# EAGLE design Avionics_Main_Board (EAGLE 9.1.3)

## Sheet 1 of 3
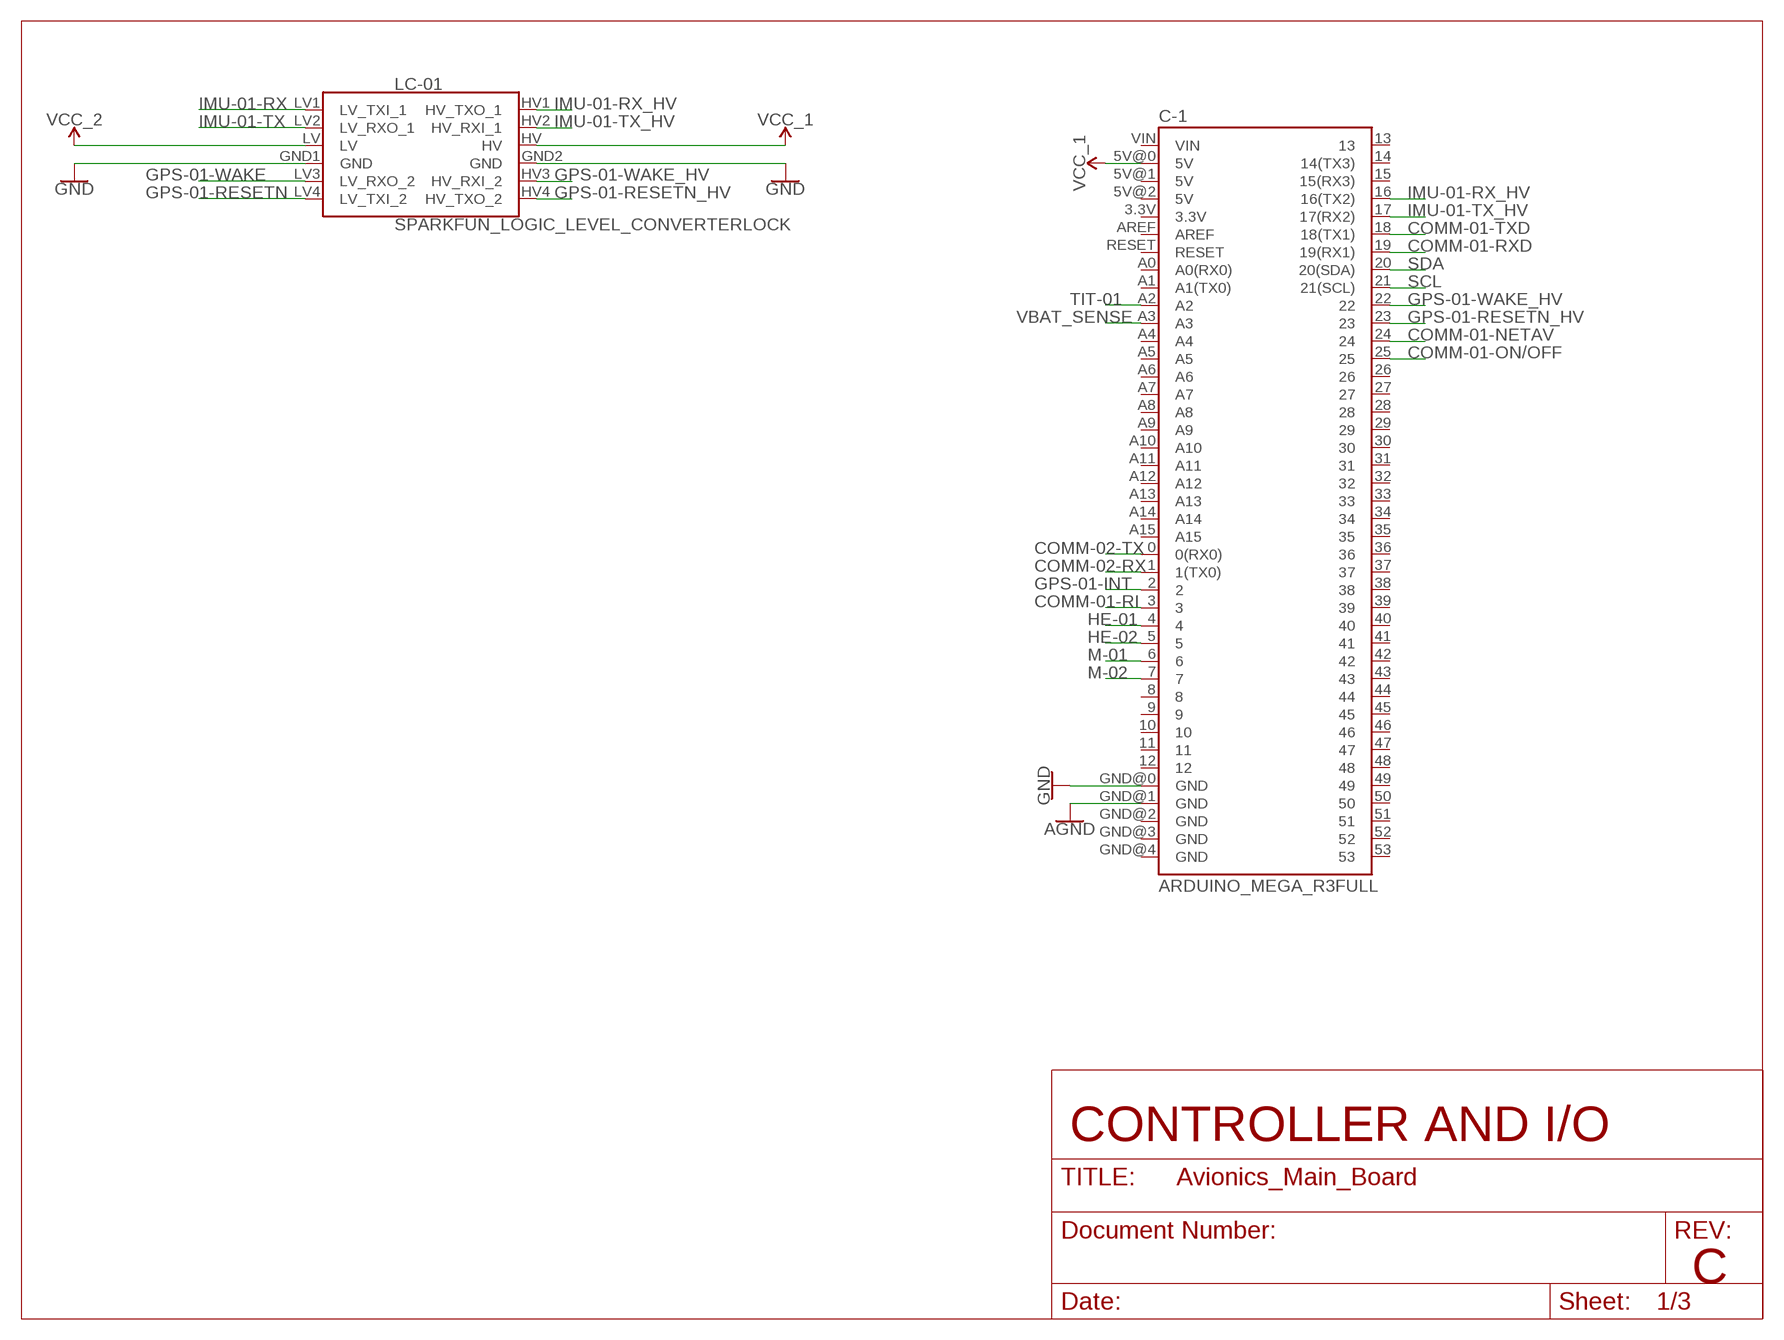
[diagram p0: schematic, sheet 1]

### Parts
C-1  ARDUINO_MEGA_R3FULL  [ARDUINO_MEGA]
LC-01  SPARKFUN_LOGIC_LEVEL_CONVERTERLOCK  [SPARKFUN_LOGIC_LEVEL_CONVERTER_LOCK]

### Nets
AGND: C-1.GND@1(GND) ; also sheet 3
COMM-01-NETAV: C-1.24 ; also sheet 3
COMM-01-ON/OFF: C-1.25 ; also sheet 3
COMM-01-RI: C-1.3 ; also sheet 3
COMM-01-RXD: C-1.19(19(RX1)) ; also sheet 3
COMM-01-TXD: C-1.18(18(TX1)) ; also sheet 3
COMM-02-RX: C-1.1(1(TX0)) ; also sheet 3
COMM-02-TX: C-1.0(0(RX0)) ; also sheet 3
GND: C-1.GND@0(GND) LC-01.GND1(GND) LC-01.GND2(GND) ; also sheet 2,3
GPS-01-INT: C-1.2 ; also sheet 3
GPS-01-RESETN: LC-01.LV4(LV_TXI_2) ; also sheet 3
GPS-01-RESETN_HV: C-1.23 LC-01.HV4(HV_TXO_2)
GPS-01-WAKE: LC-01.LV3(LV_RXO_2) ; also sheet 3
GPS-01-WAKE_HV: C-1.22 LC-01.HV3(HV_RXI_2)
HE-01: C-1.4 ; also sheet 2
HE-02: C-1.5 ; also sheet 2
IMU-01-RX: LC-01.LV1(LV_TXI_1) ; also sheet 3
IMU-01-RX_HV: C-1.16(16(TX2)) LC-01.HV1(HV_TXO_1)
IMU-01-TX: LC-01.LV2(LV_RXO_1) ; also sheet 3
IMU-01-TX_HV: C-1.17(17(RX2)) LC-01.HV2(HV_RXI_1)
M-01: C-1.6 ; also sheet 2
M-02: C-1.7 ; also sheet 2
SCL: C-1.21(21(SCL)) ; also sheet 3
SDA: C-1.20(20(SDA)) ; also sheet 3
TIT-01: C-1.A2 ; also sheet 3
VBAT_SENSE: C-1.A3 ; also sheet 3
VCC_1 [power]: C-1.5V@0(5V) LC-01.HV ; also sheet 2,3
VCC_2 [power]: LC-01.LV ; also sheet 2,3
Unconnected: C-1.3.3V C-1.5V@1(5V) C-1.5V@2(5V) C-1.8 C-1.9 C-1.10 C-1.11 C-1.12 C-1.13 C-1.14(14(TX3)) C-1.15(15(RX3)) C-1.26 C-1.27 C-1.28 C-1.29 C-1.30 C-1.31 C-1.32 C-1.33 C-1.34 C-1.35 C-1.36 C-1.37 C-1.38 C-1.39 C-1.40 C-1.41 C-1.42 C-1.43 C-1.44 C-1.45 C-1.46 C-1.47 C-1.48 C-1.49 C-1.50 C-1.51 C-1.52 C-1.53 C-1.A0(A0(RX0)) C-1.A1(A1(TX0)) C-1.A4 C-1.A5 C-1.A6 C-1.A7 C-1.A8 C-1.A9 C-1.A10 C-1.A11 C-1.A12 C-1.A13 C-1.A14 C-1.A15 C-1.AREF C-1.GND@2(GND) C-1.GND@3(GND) C-1.GND@4(GND) C-1.RESET C-1.VIN

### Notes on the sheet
- CONTROLLER AND I/O
- C

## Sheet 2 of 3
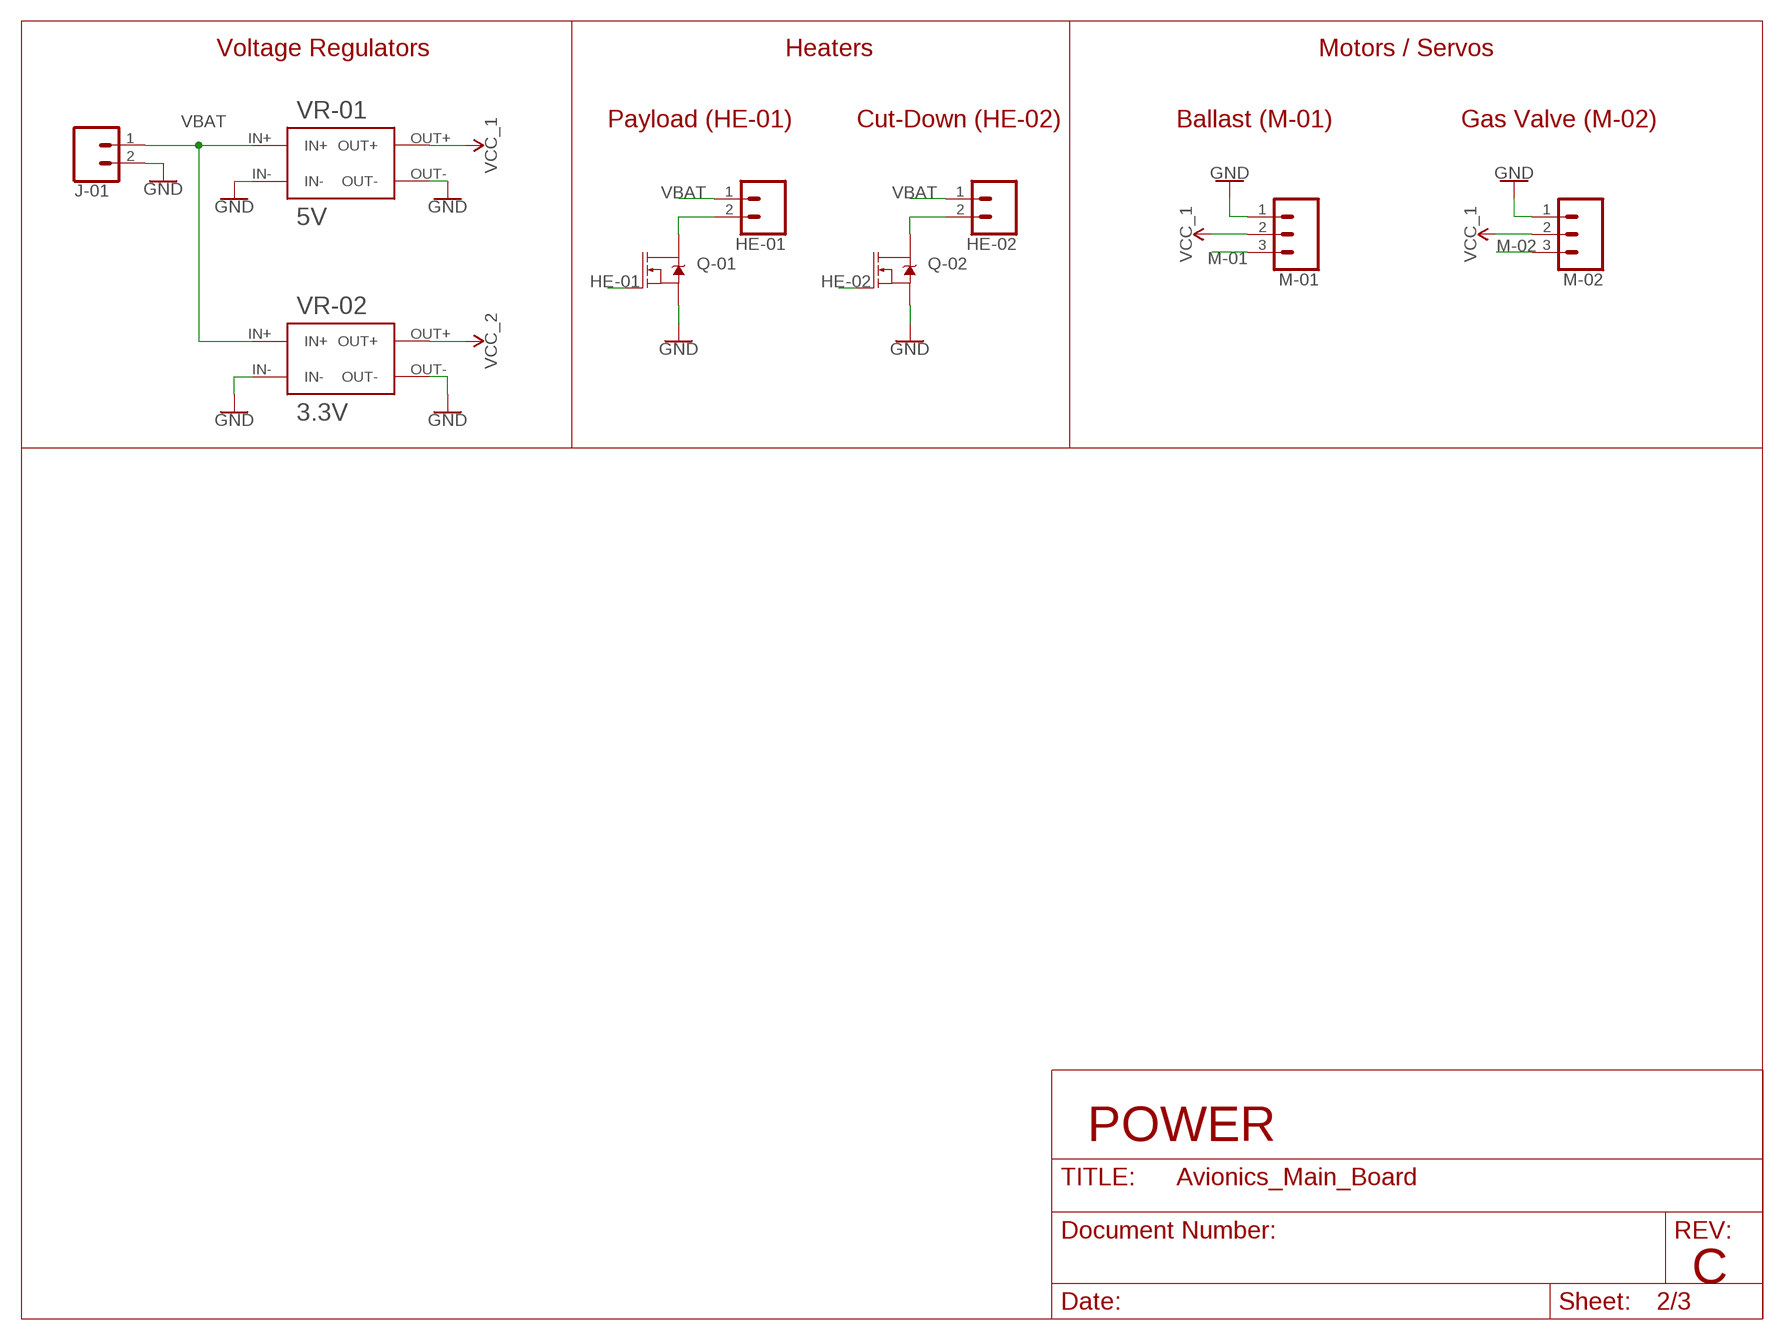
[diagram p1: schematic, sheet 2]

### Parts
HE-01  CONN_02LOCK  [1X02_LOCK]
HE-02  CONN_02LOCK  [1X02_LOCK]
J-01  CONN_023.5MM_LOCK  [SCREWTERMINAL-3.5MM-2_LOCK]
M-01  CONN_03LOCK  [1X03_LOCK]
M-02  CONN_03LOCK  [1X03_LOCK]
Q-01  MOSFET-NCH-FQP30N06L  [TO220V]
Q-02  MOSFET-NCH-FQP30N06L  [TO220V]
VR-01  5V  RIORAND_LM2596_BREAKOUT  [RIORAND_LM2596_BREAKOUT]
VR-02  3.3V  RIORAND_LM2596_BREAKOUT  [RIORAND_LM2596_BREAKOUT]

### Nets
GND: J-01.2 M-01.1 M-02.1 Q-01.3(S) Q-02.3(S) VR-01.IN- VR-01.OUT- VR-02.IN- VR-02.OUT- ; also sheet 1,3
HE-01: Q-01.1(G) ; also sheet 1
HE-01_OUT [power]: HE-01.2 Q-01.2(D)
HE-02: Q-02.1(G) ; also sheet 1
HE-02_OUT [power]: HE-02.2 Q-02.2(D)
M-01: M-01.3 ; also sheet 1
M-02: M-02.3 ; also sheet 1
VBAT [power]: HE-01.1 HE-02.1 J-01.1 VR-01.IN+ VR-02.IN+ ; also sheet 3
VCC_1 [power]: M-01.2 M-02.2 VR-01.OUT+ ; also sheet 1,3
VCC_2 [power]: VR-02.OUT+ ; also sheet 1,3

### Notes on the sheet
- Voltage Regulators | Heaters | Motors / Servos
- Payload (HE-01) | Cut-Down (HE-02) | Ballast (M-01) | Gas Valve (M-02)
- POWER
- C

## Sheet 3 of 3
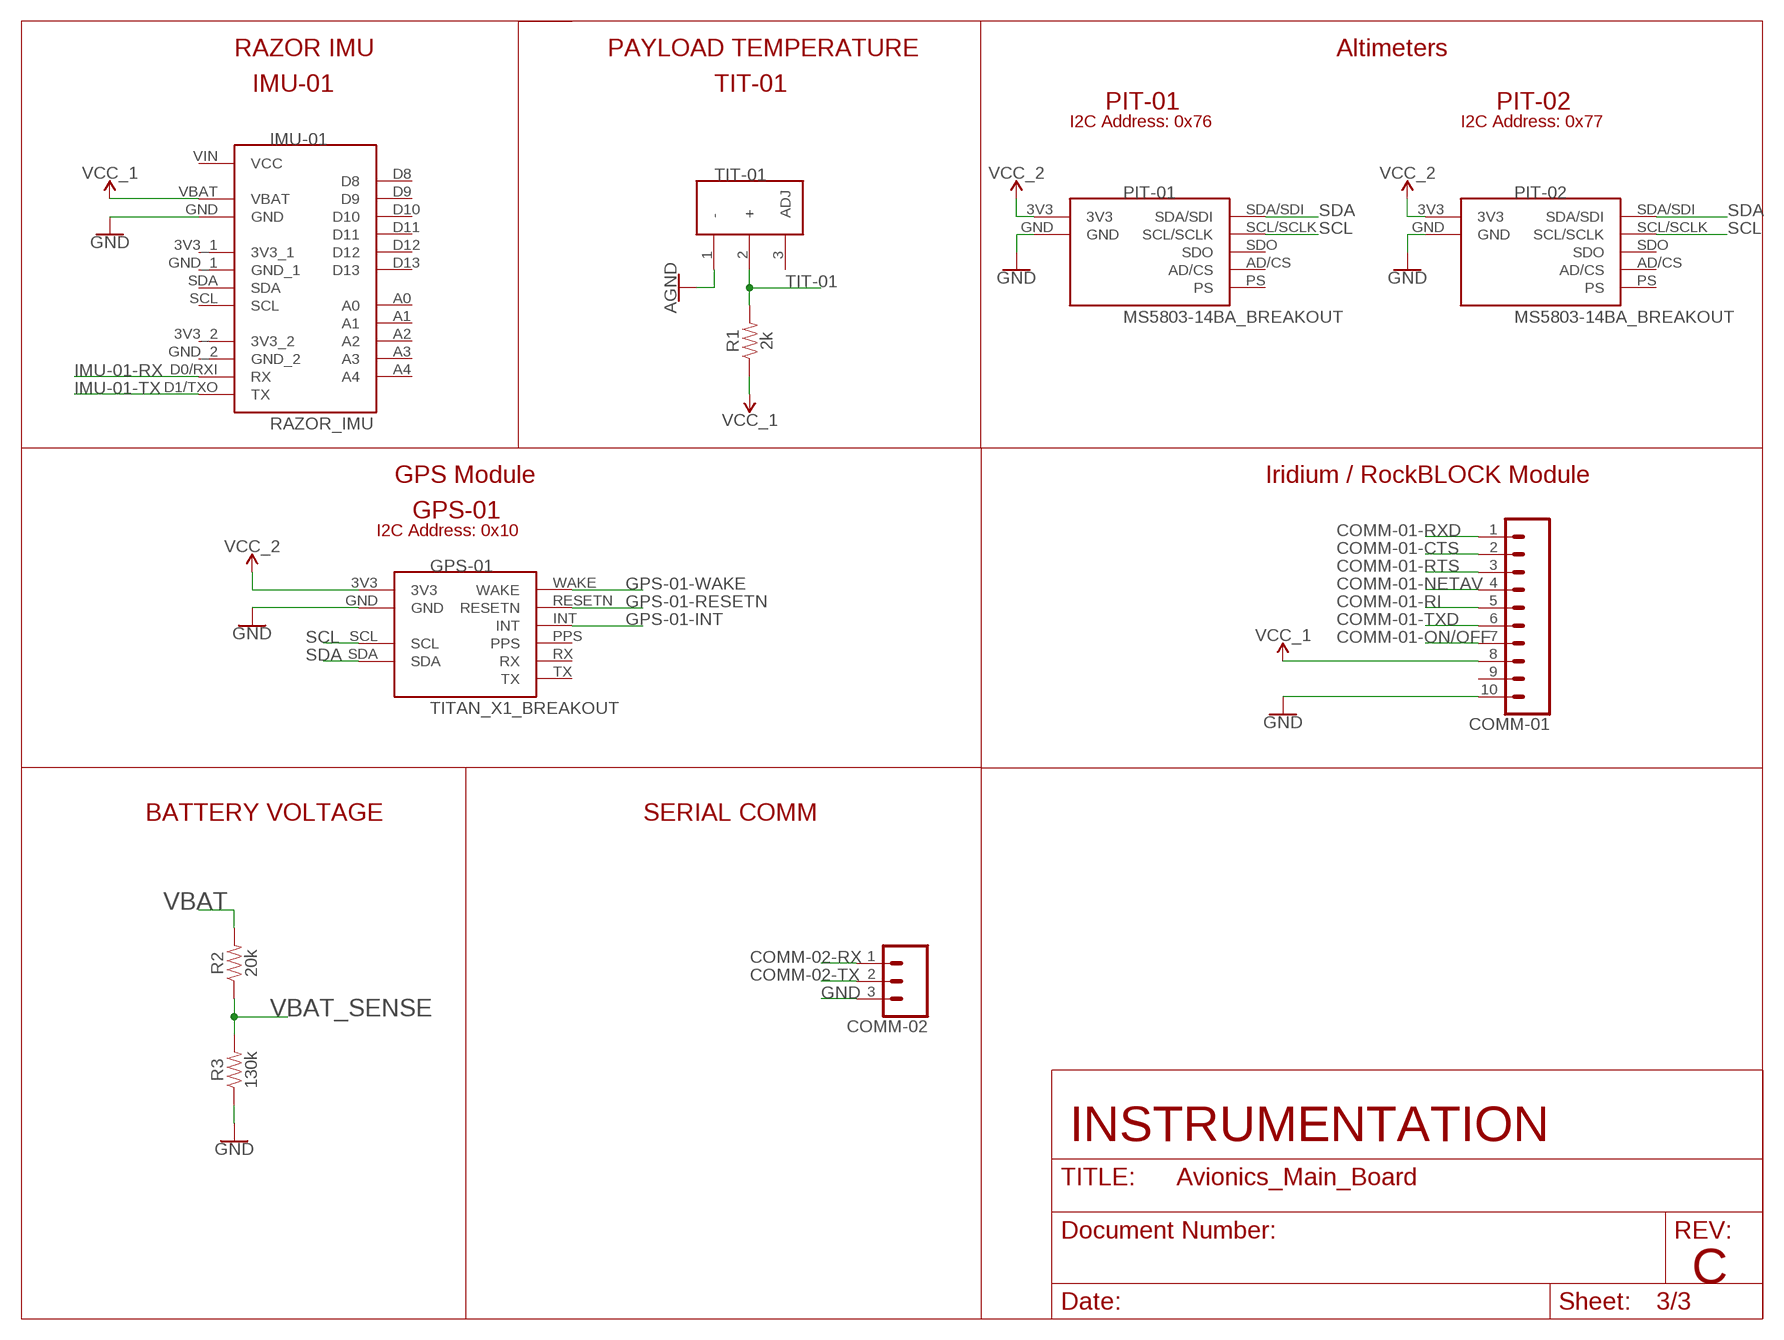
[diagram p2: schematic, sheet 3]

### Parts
COMM-01  CONN_10"  [1X10]
COMM-02  CONN_03LOCK  [1X03_LOCK]
GPS-01  TITAN_X1_BREAKOUT  [QWIIC_TITAN_X1_BREAKOUT]
IMU-01  RAZOR_IMU  [RAZOR_IMU]
PIT-01  MS5803-14BA_BREAKOUT  [MS5803-14BA_BREAKOUT]
PIT-02  MS5803-14BA_BREAKOUT  [MS5803-14BA_BREAKOUT]
R1  2k  1KOHM-HORIZ-1/4W-5%  [AXIAL-0.3]
R2  20k  1KOHM-HORIZ-1/4W-5%  [AXIAL-0.3]
R3  130k  1KOHM-HORIZ-1/4W-5%  [AXIAL-0.3]
TIT-01  LM335TO-92  [TO92]

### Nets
AGND: TIT-01.1(-) ; also sheet 1
COMM-01-CTS: COMM-01.2
COMM-01-NETAV: COMM-01.4 ; also sheet 1
COMM-01-ON/OFF: COMM-01.7 ; also sheet 1
COMM-01-RI: COMM-01.5 ; also sheet 1
COMM-01-RTS: COMM-01.3
COMM-01-RXD: COMM-01.1 ; also sheet 1
COMM-01-TXD: COMM-01.6 ; also sheet 1
COMM-02-RX: COMM-02.1 ; also sheet 1
COMM-02-TX: COMM-02.2 ; also sheet 1
GND: COMM-01.10 COMM-02.3 GPS-01.GND IMU-01.GND PIT-01.GND PIT-02.GND R3.P$1 ; also sheet 1,2
GPS-01-INT: GPS-01.INT ; also sheet 1
GPS-01-RESETN: GPS-01.RESETN ; also sheet 1
GPS-01-WAKE: GPS-01.WAKE ; also sheet 1
IMU-01-RX: IMU-01.D0/RXI(RX) ; also sheet 1
IMU-01-TX: IMU-01.D1/TXO(TX) ; also sheet 1
SCL: GPS-01.SCL PIT-01.SCL/SCLK PIT-02.SCL/SCLK ; also sheet 1
SDA: GPS-01.SDA PIT-01.SDA/SDI PIT-02.SDA/SDI ; also sheet 1
TIT-01: R1.P$2 TIT-01.2(+) ; also sheet 1
VBAT [power]: R2.P$2 ; also sheet 2
VBAT_SENSE: R2.P$1 R3.P$2 ; also sheet 1
VCC_1 [power]: COMM-01.8 IMU-01.VBAT R1.P$1 ; also sheet 1,2
VCC_2 [power]: GPS-01.3V3 PIT-01.3V3 PIT-02.3V3 ; also sheet 1,2
Unconnected: COMM-01.9 GPS-01.PPS GPS-01.RX GPS-01.TX IMU-01.3V3_1 IMU-01.3V3_2 IMU-01.A0 IMU-01.A1 IMU-01.A2 IMU-01.A3 IMU-01.A4 IMU-01.D8 IMU-01.D9 IMU-01.D10 IMU-01.D11 IMU-01.D12 IMU-01.D13 IMU-01.GND_1 IMU-01.GND_2 IMU-01.SCL IMU-01.SDA IMU-01.VIN(VCC) PIT-01.AD/CS PIT-01.PS PIT-01.SDO PIT-02.AD/CS PIT-02.PS PIT-02.SDO TIT-01.3(ADJ)

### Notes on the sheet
- RAZOR IMU | PAYLOAD TEMPERATURE | Altimeters
- IMU-01 | TIT-01
- PIT-01 | PIT-02
- I2C Address: 0x76 | I2C Address: 0x77
- GPS Module | Iridium / RockBLOCK Module
- GPS-01
- I2C Address: 0x10
- BATTERY VOLTAGE | SERIAL COMM
- INSTRUMENTATION
- C

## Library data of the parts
C-1 = SparkFun-Boards:ARDUINO_MEGA_R3: Arduino Mega R3 ATmega2560 R3 compatible footprint. SparkFun Products: Arduino Mega 2560 R3
COMM-01 = SparkFun-Connectors:CONN_10: Multi connection point. Often used as Generic Header-pin footprint for 0.1 inch spaced/style header connections On any of the 0.1 inch spaced packages, you can populate with these: Break Away Headers - Straight (PRT-00116) Break Away Male Headers - Right Angle (PRT-00553) Female Headers (PRT-00115)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; PROD_ID: CONN-11563
COMM-02 M-01 M-02 = SparkFun-Connectors:CONN_03: Multi connection point. Often used as Generic Header-pin footprint for 0.1 inch spaced/style header connections On any of the 0.1 inch spaced packages, you can populate with these: Break Away Headers - Straight (PRT-00116) Break Away Male Headers - Right Angle (PRT-00553) Female Headers (PRT-00115)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
GPS-01 = High Ball Library:TITAN_X1_BREAKOUT
HE-01 HE-02 = SparkFun-Connectors:CONN_02: Multi connection point. Often used as Generic Header-pin footprint for 0.1 inch spaced/style header connections
IMU-01 = High Ball Library:RAZOR_IMU
J-01 = SparkFun-Connectors:CONN_02: Multi connection point. Often used as Generic Header-pin footprint for 0.1 inch spaced/style header connections; PROD_ID: CONN-08399
LC-01 = SparkFun-Boards:SPARKFUN_LOGIC_LEVEL_CONVERTER: SparkFun Logic Level Converter -Bi-Directional This is the mechnical outline for the 3.3V - 5V bi directional logic level converter. *Note, the "LOCK" Package has the header pins staggered by an offset of 5 mils (off center line), so that when you slide a row of standard 0.1" headers into the PTH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
PIT-01 PIT-02 = High Ball Library:MS5803-14BA_BREAKOUT
Q-01 Q-02 = SparkFun-DiscreteSemi:MOSFET-NCH: N-channel MOSFETs Voltage controlled devices that allow control of high current outputs. SparkFun Products: SparkFun OpenScale SparkFun Digital Sandbox SparkFun Monster Moto Shield SparkFun MOSFET Power Controller; PROD_ID: TRANS-10060; VALUE: 60V/32A/35mΩ
R1-R3 = SparkFun-Resistors:1KOHM: 1kΩ resistor; PROD_ID: RES-08380; VALUE: 1k
TIT-01 = High Ball Library:LM335
VR-01 VR-02 = High Ball Library:RIORAND_LM2596_BREAKOUT

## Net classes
0 default: width 0.635 mm, drill 0.899 mm, clearance 0.381 mm
1 power: width 1.016 mm, drill 0.899 mm, clearance 0.762 mm

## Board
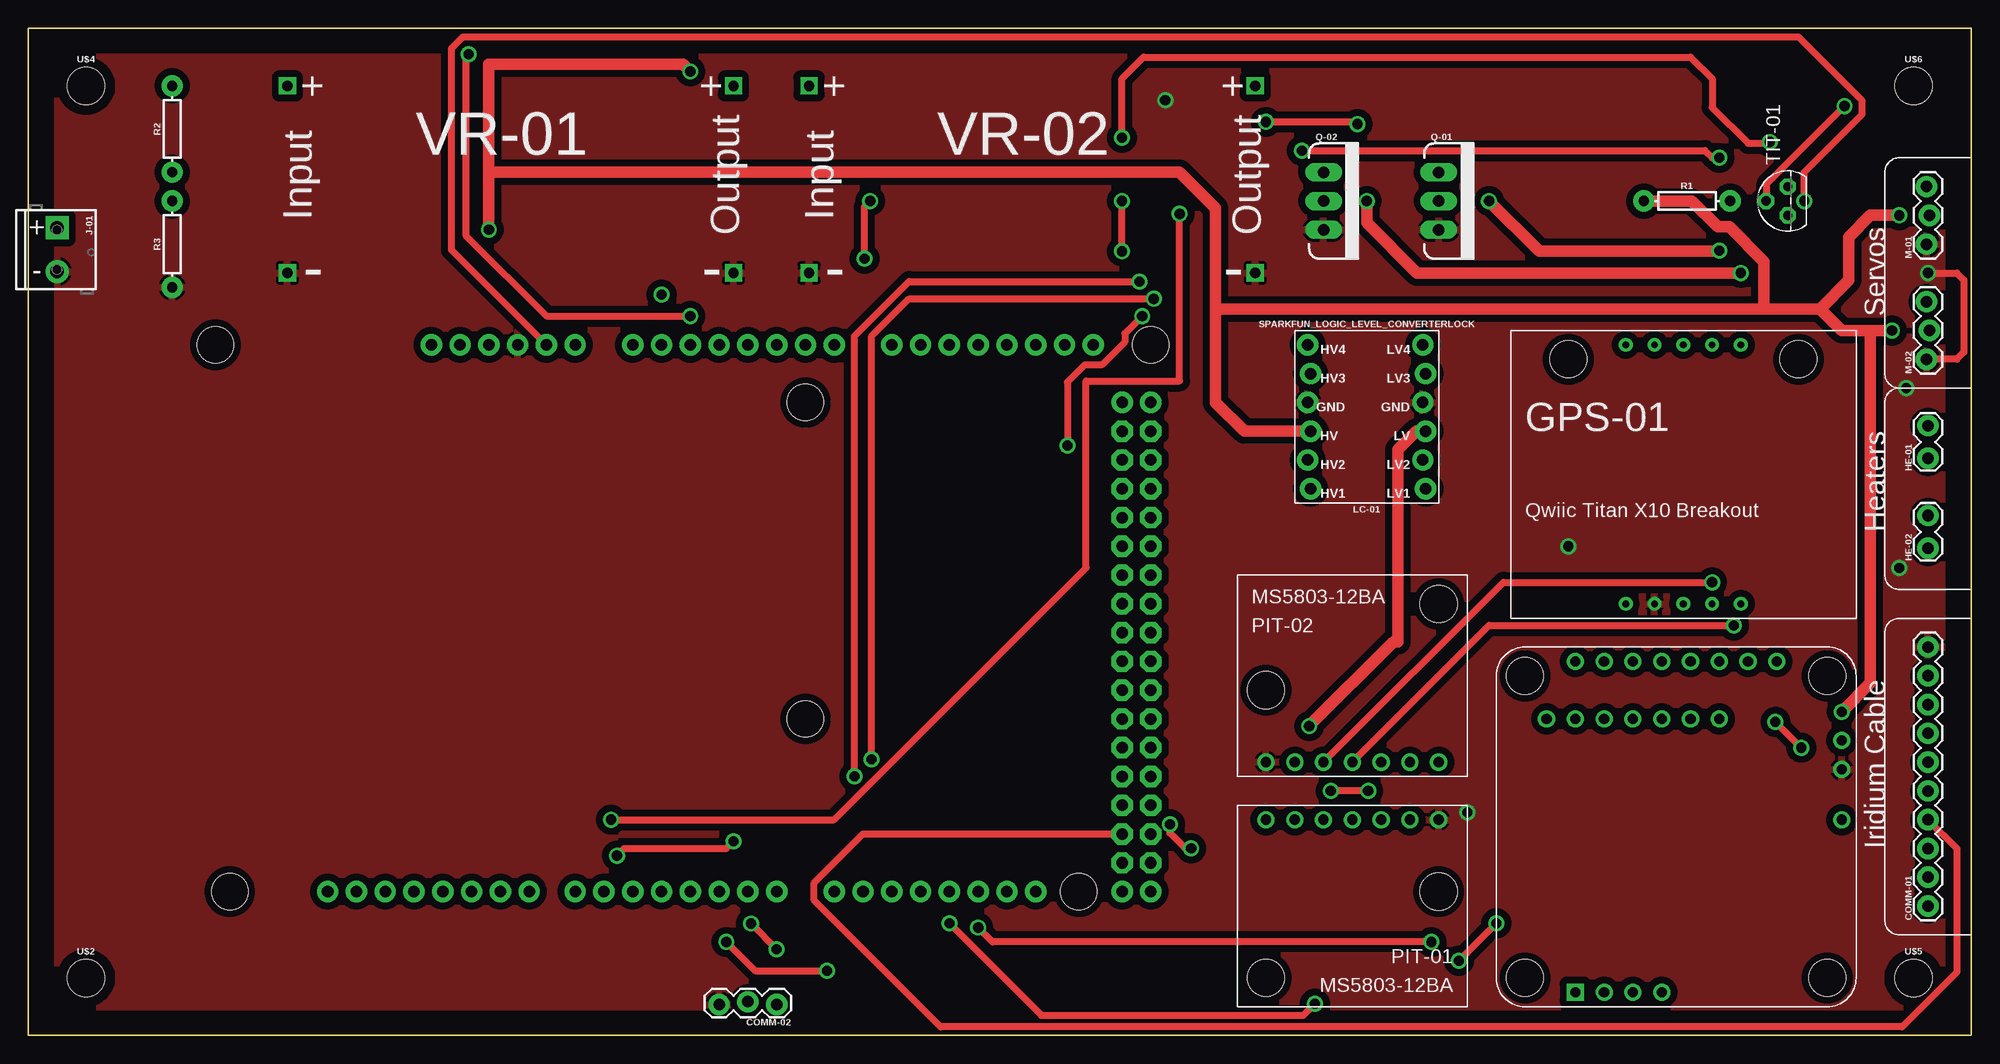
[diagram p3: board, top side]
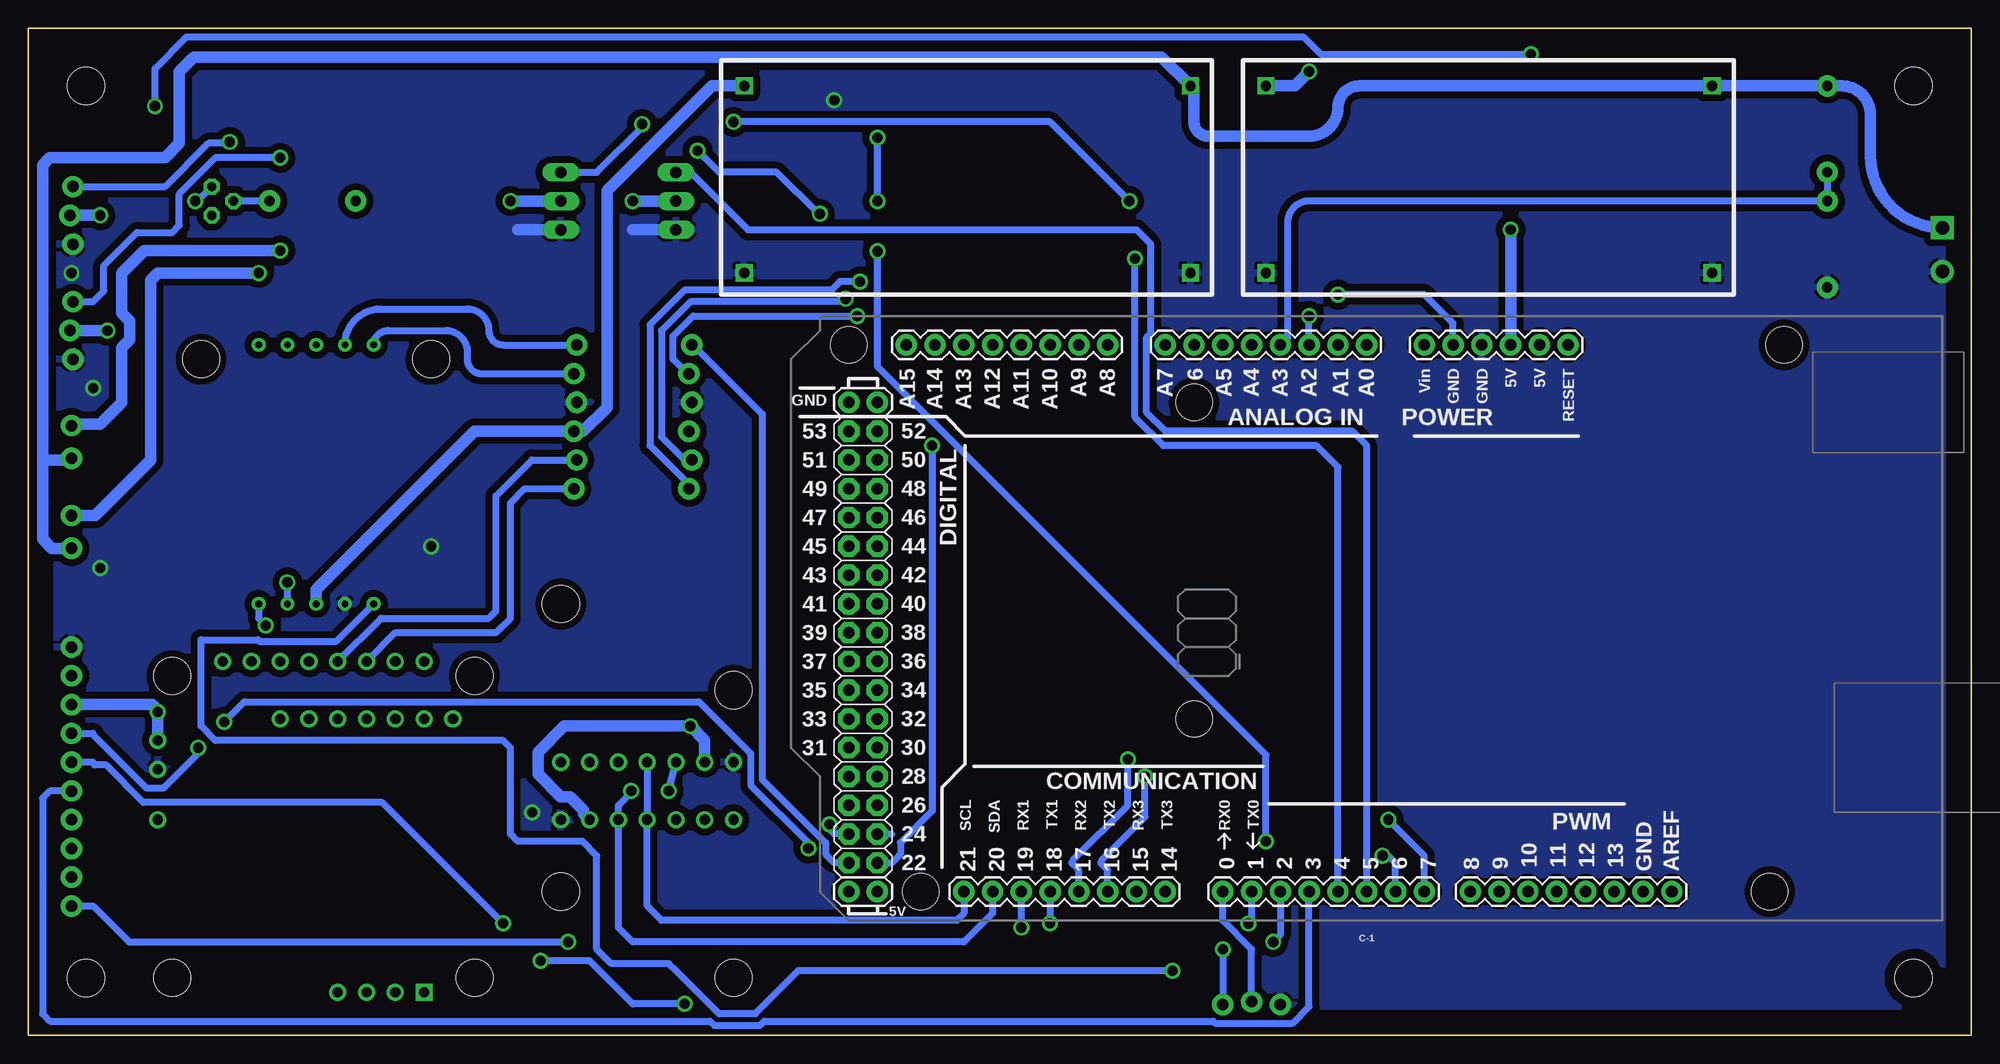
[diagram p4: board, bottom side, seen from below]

Size 171.45 x 88.9 mm. Coordinates in mm from the lower left corner, seen from the top.
Outline: 0,0 171.45,0 171.45,88.9 0,88.9 0,0
Copper layers (1*16): Top 0.035mm / dielectric 1.5mm / Bottom 0.035mm
Design rules "SparkFun": minimum track width 8mil, minimum drill 20mil, track to track 8mil, track to pad 8mil, pad to pad 8mil, via to via 8mil, smd to smd 8mil, copper to edge 10mil, drill to drill 8mil, minimum pad ring 12mil, minimum via ring 10mil, stop-mask expansion 4mil, vias tented up to drill 25mil, thermal gap 10mil

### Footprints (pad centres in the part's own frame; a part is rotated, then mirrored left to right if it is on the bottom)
ARDUINO_MEGA = drill 1.016 pad 1.88: 0 13.97,24.13; 1 11.43,24.13; 2 8.89,24.13; 3 6.35,24.13; 3.3V -13.97,-24.13; 4 3.81,24.13; 5 1.27,24.13; 5V@0 -11.43,-24.13; 5V@1 44.45,24.13; 5V@2 46.99,24.13; 6 -1.27,24.13; 7 -3.81,24.13; 8 -7.874,24.13; 9 -10.414,24.13; 10 -12.954,24.13; 11 -15.494,24.13; 12 -18.034,24.13; 13 -20.574,24.13; 14 19.05,24.13; 15 21.59,24.13; 16 24.13,24.13; 17 26.67,24.13; 18 29.21,24.13; 19 31.75,24.13; 20 34.29,24.13; 21 36.83,24.13; A0 1.27,-24.13; A1 3.81,-24.13; A2 6.35,-24.13; A3 8.89,-24.13; A4 11.43,-24.13; A5 13.97,-24.13; A6 16.51,-24.13; A7 19.05,-24.13; A8 24.13,-24.13; A9 26.67,-24.13; A10 29.21,-24.13; A11 31.75,-24.13; A12 34.29,-24.13; A13 36.83,-24.13; A14 39.37,-24.13; A15 41.91,-24.13; AREF -25.654,24.13; GND@0 -8.89,-24.13; GND@1 -6.35,-24.13; GND@2 44.45,-19.05; GND@3 46.99,-19.05; GND@4 -23.114,24.13; RESET -16.51,-24.13; VIN -3.81,-24.13 | drill 1.016 pad 1.88 octagon: 22 44.45,21.59; 23 46.99,21.59; 24 44.45,19.05; 25 46.99,19.05; 26 44.45,16.51; 27 46.99,16.51; 28 44.45,13.97; 29 46.99,13.97; 30 44.45,11.43; 31 46.99,11.43; 32 44.45,8.89; 33 46.99,8.89; 34 44.45,6.35; 35 46.99,6.35; 36 44.45,3.81; 37 46.99,3.81; 38 44.45,1.27; 39 46.99,1.27; 40 44.45,-1.27; 41 46.99,-1.27; 42 44.45,-3.81; 43 46.99,-3.81; 44 44.45,-6.35; 45 46.99,-6.35; 46 44.45,-8.89; 47 46.99,-8.89; 48 44.45,-11.43; 49 46.99,-11.43; 50 44.45,-13.97; 51 46.99,-13.97; 52 44.45,-16.51; 53 46.99,-16.51 | hole 3.2: -34.29,24.13; -35.56,-24.13; 16.51,8.89; 16.51,-19.05; 40.64,24.13; 46.99,-24.13
1X10 = drill 1.016 pad 1.88: 1 0,0; 2 2.54,0; 3 5.08,0; 4 7.62,0; 5 10.16,0; 6 12.7,0; 7 15.24,0; 8 17.78,0; 9 20.32,0; 10 22.86,0
1X03_LOCK = drill 1.016 pad 1.88: 1 0,0.127; 2 2.54,-0.127; 3 5.08,0.127
QWIIC_TITAN_X1_BREAKOUT = drill 0.6: 3V3 15.24,1.27; GND 12.7,1.27; INT 10.16,1.27; PPS 15.24,24.13; RESETN 12.7,24.13; RX 17.78,24.13; SCL 20.32,1.27; SDA 17.78,1.27; TX 20.32,24.13; WAKE 10.16,24.13 | hole 3.264: 5.08,22.86; 25.4,22.86
1X02_LOCK = drill 1.016 pad 1.88: 1 -0.178,0; 2 2.718,0
RAZOR_IMU = drill 0.9: 3V3_1 1.27,22.225; 3V3_2 30.48,22.225; A0 25.4,12.065; A1 25.4,14.605; A2 25.4,17.145; A3 25.4,19.685; A4 25.4,22.225; D0/RXI 30.48,19.685; D1/TXO 30.48,17.145; D8 25.4,24.765; D9 25.4,27.305; D10 30.48,14.605; D11 30.48,12.065; D12 30.48,9.525; D13 30.48,6.985; GND 20.955,1.27; GND_2 30.48,24.765; SCL 1.27,17.145; SDA 1.27,19.685; VBAT 23.495,1.27; VIN 16.51,1.27 | drill 0.9 square: GND_1 1.27,24.765 | hole 3.264: 2.54,2.54; 29.21,2.54; 29.21,29.21; 2.54,29.21
SCREWTERMINAL-3.5MM-2_LOCK = drill 1.2 pad 2.032 square: 1 -0.178,0 | drill 1.2 pad 2.032: 2 3.678,0
SPARKFUN_LOGIC_LEVEL_CONVERTER_LOCK = drill 1.016 pad 1.88: GND1 -4.953,-1.27; GND2 5.207,-1.27; HV 4.953,1.27; HV1 4.953,6.35; HV2 5.207,3.81; HV3 4.953,-3.81; HV4 5.207,-6.35; LV -5.207,1.27; LV1 -5.207,6.35; LV2 -4.953,3.81; LV3 -5.207,-3.81; LV4 -4.953,-6.35
MS5803-14BA_BREAKOUT = drill 0.9: 3V3 5.08,1.27; AD/CS 15.24,1.27; GND 2.54,1.27; PS 17.78,1.27; SCL/SCLK 10.16,1.27; SDA/SDI 7.62,1.27; SDO 12.7,1.27 | hole 3.264: 17.78,15.24; 2.54,7.62
TO220V = drill 1.016 long: 1 -2.54,0; 2 0,0; 3 2.54,0
AXIAL-0.3 = drill 0.9 pad 1.88: P$1 -3.81,0; P$2 3.81,0
TO92 = drill 0.813 octagon: 1 1.27,0; 2 0,1.905; 3 -1.27,0
STAND-OFF = hole 3.302: 0,0
RIORAND_LM2596_BREAKOUT = drill 0.9 square: IN+ 0,16.51; IN- 0,0; OUT+ 39.37,16.51; OUT- 39.37,0

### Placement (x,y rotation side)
C-1  52.07,36.83 180 bottom
COMM-01  167.64,11.43 90 top
COMM-02  66.04,2.86 180 top
GPS-01  130.81,36.83 0 top
HE-01  167.64,51.12 90 top
HE-02  167.64,43.18 90 top
IMU-01  161.29,2.54 90 top
J-01  2.54,71.12 270 top
LC-01  118.11,54.61 180 top
M-01  167.64,69.85 90 top
M-02  167.64,59.69 90 top
PIT-01  127,20.32 180 top
PIT-02  106.68,22.86 0 top
Q-01  124.46,73.66 270 top
Q-02  114.3,73.66 270 top
R1  146.37,73.66 0 top
R2  12.7,80.01 90 top
R3  12.7,69.85 90 top
TIT-01  155.26,73.66 90 top
U$2  [STAND-OFF]  5.08,5.08 0 top
U$4  [STAND-OFF]  5.08,83.82 0 top
U$5  [STAND-OFF]  166.37,5.08 0 top
U$6  [STAND-OFF]  166.37,83.82 0 top
VR-01  22.86,67.31 0 top
VR-02  68.9,67.31 0 top

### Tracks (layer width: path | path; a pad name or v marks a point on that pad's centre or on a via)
AGND  (via drill 0.9)
  Top 0.635: C-1.GND@1 37.34,69.34 37.34,87.12 38.35,88.14 156.21,88.14 161.8,82.55 161.8,81.28 156.78,76.26 156.71,76.19 v156.71,73.66
  Bottom 0.635: C-1.GND@1 45.72,62.87 48.26,65.41 v55.88,65.41 | TIT-01.1 156.53,73.66 v156.71,73.66 156.84,73.66
COMM-01-NETAV
  Top 0.635: C-1.24 73.66,17.78 69.34,13.46 69.34,11.94 80.52,0.76 165.35,0.76 170.18,5.59 170.18,16.51 COMM-01.4
  Bottom 0.635: C-1.24 95.25,17.78
COMM-01-ON/OFF  (via drill 0.9)
  Top 0.635: v102.62,16.51 102.11,16.51 100.74,17.88 v100.74,18.64 | v156.46,25.4 v154.18,27.69
  Bottom 0.635: COMM-01.7 165.74,26.67 165.61,26.42 161.04,21.84 159.51,21.84 156.46,24.89 v156.46,25.4 | C-1.25 100.33,17.78 100.74,18.19 v100.74,18.64 | v102.62,16.51 102.62,17.02 107.7,22.1 107.7,24.89 112.27,29.46 152.4,29.46 v154.18,27.69
COMM-01-RI
  Bottom 0.635: COMM-01.5 169.54,21.59 170.18,20.95 170.18,1.91 169.54,1.27 111.29,1.27 110.91,0.89 106.89,0.89 106.51,1.27 66.9,1.27 66.72,1.09 59.87,1.09 58.42,2.54 C-1.3
COMM-01-RXD  (via drill 0.9)
  Top 0.635: v123.83,8.26 85.09,8.26 v83.82,9.53
  Bottom 0.635: COMM-01.1 165.74,11.43 162.56,8.26 v123.83,8.26 | v83.82,9.53 C-1.19
COMM-01-TXD  (via drill 0.9)
  Top 0.635: v126.24,6.6 v129.54,9.91 | v113.54,2.79 112.52,1.78 89.41,1.78 v81.28,9.91
  Bottom 0.635: COMM-01.6 165.74,24.13 165.61,23.88 164.59,23.88 161.29,20.57 140.21,20.57 v129.54,9.91 | v126.24,6.6 121.92,6.6 118.11,2.79 v113.54,2.79 | C-1.18 v81.28,9.91
COMM-02-RX  (via drill 0.9)
  Top 0.635: v63.78,9.88 v66.04,7.62
  Bottom 0.635: C-1.1 63.5,10.16 v63.78,9.88 | v66.04,7.62 COMM-02.1
COMM-02-TX
  Bottom 0.635: C-1.0 66.04,10.16 63.5,7.62 COMM-02.2
GND  (via drill 0.9)
  Top 0.635: v167.64,67.31 170.18,67.31 170.8,66.69 170.8,60.31 170.18,59.69 M-02.1
  Bottom 1.016: Q-02.3 118.11,71.12 | Q-01.3 128.27,71.12
  other vias: 135.89,43.18 127,19.68 100.33,82.55 165.1,41.27 165.74,57.15
  pour Top (isolate 0.61): 2.54,2.54 168.91,2.54 168.91,86.36 2.54,86.36
  pour Bottom (isolate 0.61): 2.54,2.54 168.91,2.54 168.91,86.36 2.54,86.36
GPS-01-INT  (via drill 0.9)
  Top 0.635: v61.59,8.26 64.14,5.71 v70.48,5.71
  Bottom 0.635: v61.59,8.26 60.96,8.89 C-1.2 | v70.48,5.71 103.5,5.71 | 103.5,5.71 | 103.5,5.71 107.31,1.91 110.49,1.91 114.3,5.71 114.94,6.35 120.02,6.35 121.28,7.62 121.28,15.88 122.56,17.14 128.27,17.14 128.91,17.78 128.91,25.4 129.54,26.04 154.94,26.04 156.21,27.3 156.21,34.92 151.21,34.92 151.08,34.79 144.28,34.79 GPS-01.INT
GPS-01-RESETN
  Bottom 0.635: GPS-01.RESETN arc90 140.34,64.14 132.72,64.14 arc90 130.81,62.23 arc-90 129.54,60.96 LC-01.LV4
GPS-01-RESETN_HV
  Bottom 0.635: C-1.23 100.33,15.24 100.97,15.88 101.09,16 101.09,17.02 106.68,22.61 106.68,54.86 112.78,60.96 LC-01.HV4
GPS-01-WAKE
  Bottom 0.635: GPS-01.WAKE arc90 139.7,62.23 134.62,62.23 arc90 132.72,60.33 132.72,59.69 arc-90 131.44,58.42 LC-01.LV3
GPS-01-WAKE_HV  (via drill 0.9)
  Top 0.635: v91.69,52.07 91.69,57.66 93.22,59.18 94.74,59.18 96.77,61.21 96.77,61.98 v98.3,63.5
  Bottom 0.635: C-1.22 95.25,15.24 94.61,15.88 94.49,16 94.49,17.02 91.69,19.81 v91.69,52.07 | v98.3,63.5 112.78,63.5 114.55,61.72 114.55,59.69 113.28,58.42 LC-01.HV3
HE-01  (via drill 0.9)
  Top 0.635: v73.79,68.58 73.79,73.16 v74.3,73.66 | v117.28,80.45 117.09,80.64 v109.22,80.64
  Bottom 0.635: C-1.4 55.88,14.61 | Q-01.1 121.28,76.2 | 121.28,76.2 | 121.28,76.2 117.16,80.33 v117.28,80.45 | 55.88,14.61 | 55.88,14.61 55.88,50.16 57.78,52.07 71.29,52.07 73.77,54.56 73.77,68.47 73.66,68.58 v73.79,68.58 | v74.3,73.66 81.28,80.64 v109.22,80.64
HE-01_OUT  (via drill 0.9)
  Top 1.016: v128.91,73.66 133.35,69.22 149.22,69.22 v149.22,69.28
  Bottom 1.016: Q-01.2 v128.91,73.66 | v149.22,69.28 161.22,69.28 163.19,67.31 163.19,63.75 162.49,63.05 162.49,61.41 163.19,60.71 163.19,55.88 165.1,53.98 167.5,53.98 HE-01.2
HE-02
  Bottom 0.635: Q-02.1 113.03,76.2 107.95,71.12 73.66,71.12 72.39,69.85 72.39,62.01 72.76,61.64 72.76,54.98 71.12,53.34 54.61,53.34 53.34,52.07 C-1.5
HE-02_OUT  (via drill 0.9)
  Top 1.016: v118.11,73.66 118.11,71.75 122.56,67.31 v151.13,67.31
  Bottom 1.016: Q-02.2 v118.11,73.66 | HE-02.2 165.56,45.9 160.66,50.8 160.66,66.67 160.02,67.31 v151.13,67.31
IMU-01-RX
  Bottom 0.635: IMU-01.D0/RXI 139.06,35.56 130.18,35.56 128.91,36.83 128.91,46.99 127.64,48.26 LC-01.LV1
IMU-01-RX_HV  (via drill 0.9)
  Top 0.635: v98.04,66.55 77.72,66.55 72.9,61.72 v72.9,22.86
  Bottom 0.635: C-1.16 76.2,14.61 76.83,15.24 76.71,15.49 72.9,19.3 v72.9,22.86 | v98.04,66.55 99.82,66.55 100.58,65.79 113.54,65.79 116.59,62.74 116.59,52.07 113.28,48.77 113.28,48.26 LC-01.HV1
IMU-01-TX
  Bottom 0.635: IMU-01.D1/TXO 140.34,36.83 130.81,36.83 130.18,37.47 130.18,47.62 127,50.8 LC-01.LV2
IMU-01-TX_HV  (via drill 0.9)
  Top 0.635: v99.31,65.02 77.72,65.02 74.42,61.72 v74.42,24.38
  Bottom 0.635: C-1.17 78.74,14.61 79.38,15.24 79.25,15.49 74.42,20.32 v74.42,24.38 | v99.31,65.02 99.57,64.77 113.03,64.77 115.57,62.23 115.57,52.83 113.54,50.8 113.03,50.8 LC-01.HV2
M-01  (via drill 0.9)
  Top 0.635: v51.94,15.88 52.57,16.51 61.59,16.51 v62.23,17.14 | v96.52,69.22 v96.52,73.66 | v96.52,79.24 96.52,84.45 98.42,86.36 146.69,86.36 148.59,84.45 148.59,81.92 151.76,78.74 153.67,78.74 v153.67,78.87
  Bottom 0.635: M-01.3 159.38,74.93 155.57,78.74 153.67,78.74 v153.67,78.87 | v51.94,15.88 51.44,15.88 50.8,15.24 C-1.6 | v62.23,17.14 62.23,24.77 96.52,59.05 v96.52,69.22 | v96.52,73.66 v96.52,79.24
M-02  (via drill 0.9)
  Top 0.635: v101.6,72.52 101.6,57.78 93.34,57.78 93.34,41.27 71.12,19.05 v51.44,19.05 | v112.39,78.11 147.96,78.11 148.59,77.47 v149.22,77.47
  Bottom 0.635: C-1.7 48.26,14.61 | M-02.3 165.74,64.77 164.78,65.72 164.78,67.97 161.88,70.87 158.75,70.87 158.12,71.51 158.12,74.3 154.94,77.47 v149.22,77.47 | 48.26,14.61 | 48.26,14.61 48.26,15.88 v51.44,19.05 | v101.6,72.52 101.73,72.52 105.41,76.2 110.49,76.2 v112.39,78.11
SCL  (via drill 0.9)
  Top 0.635: PIT-02.SCL/SCLK 128.91,36.2 v150.5,36.2
  Bottom 0.635: GPS-01.SCL 151.13,36.83 v150.5,36.2 | PIT-02.SCL/SCLK PIT-01.SCL/SCLK 116.84,11.43 115.57,10.16 89.53,10.16 88.9,10.79 C-1.21
SDA  (via drill 0.9)
  Top 0.635: v118.24,21.59 v114.94,21.59 | PIT-02.SDA/SDI 130.18,40.01 v148.59,40.01
  Bottom 0.635: v118.24,21.59 118.11,21.59 119.38,20.32 PIT-01.SDA/SDI 119.38,9.53 118.11,8.26 88.9,8.26 86.36,10.79 C-1.20 | v114.94,21.59 PIT-02.SDA/SDI | v148.59,40.01 GPS-01.SDA
TIT-01  (via drill 0.9)
  Top 0.635: v38.86,86.61 38.61,86.36 38.61,70.61 45.72,63.5 58.17,63.5 v58.42,63.5 | v160.27,82.04 153.42,75.18 153.42,73.66 TIT-01.2
  Bottom 0.635: R1.P$2 TIT-01.2 | C-1.A2 v58.42,63.5 | v38.86,86.61 57.4,86.61 58.93,88.14 157.48,88.14 160.27,85.34 v160.27,82.04
VBAT
  Bottom 1.016: J-01.1 arc90 8.89,77.65 8.89,81.28 arc-90 11.43,83.82 R2.P$2 VR-01.IN+ 53.98,83.82 arc-90 55.88,81.92 arc90 58.42,79.38 67.31,79.38 arc90 68.58,80.64 68.58,83.5 arc-90 VR-02.IN+ 71.44,86.36 156.84,86.36 158.12,85.09 158.12,78.74 159.38,77.47 169.54,77.47 170.18,76.83 170.18,50.8 | HE-02.1 169.37,43 170.18,43.81 170.18,50.8 | 170.18,50.8 167.78,50.8 HE-01.1
VBAT_SENSE
  Bottom 0.635: C-1.A3 arc-90 60.33,61.59 60.33,71.75 arc90 58.42,73.66 R3.P$2 R2.P$1
VCC_1  (via drill 0.9)
  Top 1.016: v58.42,85.09 57.78,85.72 40.64,85.72 40.64,76.2 | v40.64,71.12 40.64,76.2 | 104.78,64.14 104.78,73.03 101.6,76.2 40.64,76.2 | 104.78,64.14 104.78,55.88 107.31,53.34 LC-01.HV | LC-01.HV 113.67,53.34 LC-01.HV | 104.78,64.14 | 104.78,64.14 153.16,64.14 | 153.16,64.14 158.12,64.14 | 158.12,64.14 160.02,62.23 162.56,62.23 | 162.56,62.23 v164.47,62.23 | 158.12,64.14 160.66,66.67 160.66,70.48 162.56,72.39 v165.1,72.39 | 162.56,62.23 162.56,31.11 v160.02,28.57 | R1.P$1 142.75,73.66 146.81,73.66 149.1,71.37 150.11,71.37 153.16,68.33 153.16,64.52 153.16,64.14
  Bottom 1.016: v58.42,85.09 59.69,83.82 VR-01.OUT+ | C-1.5V@0 v40.64,71.12 | v164.47,62.23 M-02.2 | v165.1,72.39 M-01.2 | IMU-01.VBAT v160.02,28.57 160.27,28.96 160.53,29.21 COMM-01.8
VCC_2  (via drill 0.9)
  Top 1.016: LC-01.LV 122.48,53.34 120.85,51.72 120.85,34.72 120.44,34.72 v113.03,27.3
  Bottom 1.016: VR-02.OUT+ 111.12,83.82 120.38,74.56 120.38,55.44 122.48,53.34 LC-01.LV 132.08,53.34 145.41,40.01 146.05,39.37 GPS-01.3V3 | PIT-01.3V3 122.44,19.57 122.44,19.89 123.62,21.07 124.46,21.07 126.48,23.1 126.48,24.97 124.15,27.3 v113.03,27.3 111.76,26.04 PIT-02.3V3

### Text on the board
tPlace: Servos | Heaters | Iridium Cable
tNames: + | -

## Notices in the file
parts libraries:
SparkFun-Connectors: Licensing: Creative Commons ShareAlike 4.0 International - https://creativecommons.org/licenses/by-sa/4.0
